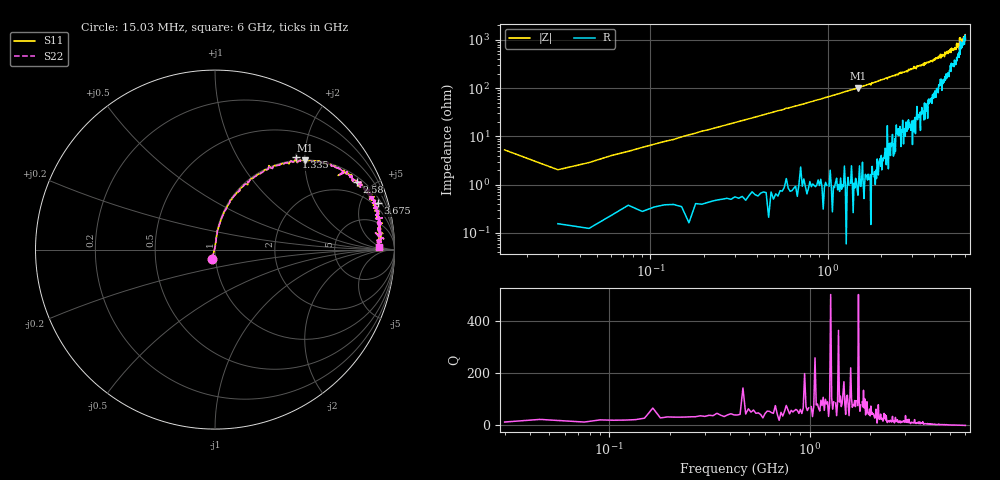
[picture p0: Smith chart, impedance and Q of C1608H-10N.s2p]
!	Network	Analyzer	HP8753E.07.74:	Oct	30	2002	Serial	No.	JP38451487
!	Hewlett-Packard
!	7	Sep	2009	10:17:20
!	Frequency	S11	S21	S12	S22
#	HZ	S	RI	R	50
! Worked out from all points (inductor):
!   400 points, 15.03 MHz to 6 GHz, reference 50 ohm
!   read as one part in series: L = 10.3 nH near 45.03 MHz
!   highest Q = 113 at 1.485 GHz (marker M1), where L = 10.8 nH
!   S11 on the Smith chart (normalised r, x): 15.03 MHz: 0.96, -0.10; 1.335 GHz: 0.94, +1.83; 2.58 GHz: 1.27, +4.05; 3.675 GHz: 1.47, +6.86; 6 GHz: 21, +3
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1.502992e7  -0.0156 -0.0503  1.02 0.0503  1.02 0.0503  -0.0156 -0.0503
3.002985e7  0.00191 0.0202  0.998 -0.0202  0.998 -0.0202  0.00191 0.0202
1.200294e8  0.00964 0.0772  0.99 -0.0772  0.99 -0.0772  0.00964 0.0772
2.850286e8  0.0372 0.176  0.963 -0.176  0.963 -0.176  0.0372 0.176
1.020025e9  0.311 0.456  0.689 -0.456  0.689 -0.456  0.311 0.456
1.335023e9  0.454 0.515  0.546 -0.515  0.546 -0.515  0.454 0.515
1.485023e9  0.504 0.497  0.496 -0.497  0.496 -0.497  0.504 0.497
2.01002e9  0.68 0.453  0.32 -0.453  0.32 -0.453  0.68 0.453
2.580017e9  0.789 0.376  0.211 -0.376  0.211 -0.376  0.789 0.376
3.015015e9  0.86 0.334  0.14 -0.334  0.14 -0.334  0.86 0.334
3.675012e9  0.907 0.258  0.0929 -0.258  0.0929 -0.258  0.907 0.258
4.00501e9  0.913 0.214  0.0871 -0.214  0.0871 -0.214  0.913 0.214
5.010005e9  0.915 0.124  0.0854 -0.124  0.0854 -0.124  0.915 0.124
5.295004e9  0.913 0.118  0.0867 -0.118  0.0867 -0.118  0.913 0.118
5.355003e9  0.935 0.0892  0.0652 -0.0892  0.0652 -0.0892  0.935 0.0892
5.535002e9  0.894 0.0928  0.106 -0.0928  0.106 -0.0928  0.894 0.0928
5.565002e9  0.94 0.0608  0.0602 -0.0608  0.0602 -0.0608  0.94 0.0608
5.595002e9  0.905 0.0826  0.0953 -0.0826  0.0953 -0.0826  0.905 0.0826
5.625002e9  0.926 0.0409  0.0744 -0.0409  0.0744 -0.0409  0.926 0.0409
5.745001e9  0.902 0.0517  0.0975 -0.0517  0.0975 -0.0517  0.902 0.0517
5.865001e9  0.924 0.0233  0.0757 -0.0233  0.0757 -0.0233  0.924 0.0233
6e9  0.911 0.0121  0.0886 -0.0121  0.0886 -0.0121  0.911 0.0121
